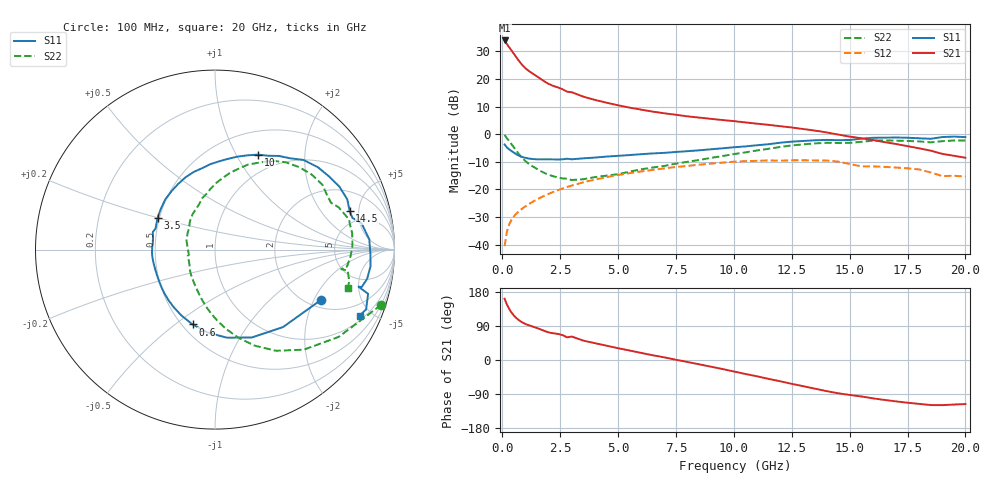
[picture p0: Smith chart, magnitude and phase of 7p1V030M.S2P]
! Infineon Technologies  Discrete & RF Semiconductors
! bfp620
! VCE =  1.0 V,  IC =  30 mA
! Common Emitter S-Parameters:  Sep 2002
# GHz  S  MA  R  50
!  f  S11  S21  S12  S22
! GHz  MAG  ANG  MAG  ANG  MAG  ANG  MAG  ANG
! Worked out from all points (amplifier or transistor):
!   59 points, 100 MHz to 20 GHz, reference 50 ohm
!   highest |S21| = 33.9 dB at 100 MHz (marker M1)
!   |S21| within 3 dB of that: start of sweep to 344.2 MHz
!   unconditionally stable (mu >= 1): 3.205 GHz to 9.953 GHz; 17.13 GHz to end of sweep
!   at 1 GHz: K = 0.78, MSG = 25.0 dB, |S12| = -26.1 dB
!   at 5.5 GHz: K = 1.04, MAG = 10.7 dB, |S12| = -14.1 dB
!   at 20 GHz: K = 1.39, MAG = -0.3 dB, |S12| = -15.3 dB
!   S11 on the Smith chart (normalised r, x): 100 MHz: 2.31, -2.26; 600 MHz: 0.56, -0.58; 3.5 GHz: 0.49, +0.20; 10 GHz: 0.77, +1.23; 14.5 GHz: 3.60, +3.96; 20 GHz: 1.25, -4.26
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0.1  0.6524 -25.6  49.83 161.6  0.0094 82.2  0.9759 -18.4
0.2  0.5745 -48.7  42.72 146.3  0.0173 70.1  0.8436 -35.2
0.3  0.531 -67.2  37.4 134.4  0.0234 65.0  0.7456 -48.4
0.4  0.4954 -82.3  32.77 125.0  0.0284 61.9  0.6584 -58.9
0.5  0.4631 -95.3  28.59 117.4  0.0325 59.7  0.578 -67.7
0.6  0.4351 -106.7  24.91 111.2  0.0362 58.2  0.5063 -75.3
0.7  0.4127 -116.7  21.79 105.9  0.0396 57.3  0.4453 -82.2
0.9  0.3828 -132.6  17.24 98.0  0.0462 56.3  0.3562 -93.6
1.1  0.3658 -143.9  14.45 92.6  0.0527 56.0  0.3009 -102.3
1.3  0.3559 -152.5  12.61 88.5  0.0594 55.6  0.2639 -109.5
2  0.3515 -177.3  8.154 72.9  0.0832 52.3  0.1846 -138.4
2.8  0.36 164.2  5.882 59.6  0.1109 46.6  0.1563 -166.7
3  0.3513 160.6  5.759 61.9  0.1177 44.9  0.1482 -168.6
3.5  0.3658 151.1  4.789 51.1  0.1347 40.4  0.153 176.1
5  0.4057 126.7  3.341 31.1  0.1826 26.1  0.1891 139.5
7  0.4598 98.7  2.391 6.9  0.2405 6.4  0.2664 109.6
10  0.5807 65.7  1.726 -30.3  0.3179 -26.8  0.4363 78.9
10.5  0.6014 60.4  1.636 -36.9  0.3254 -33.4  0.4689 73.8
13.5  0.7767 26.9  1.163 -75.6  0.3352 -69.2  0.6816 38.0
14.5  0.7803 16.0  0.986 -87.8  0.3195 -84.4  0.6941 25.6
17  0.8712 -6.2  0.665 -109.2  0.2492 -100.5  0.7656 1.4
20  0.886 -24.5  0.375 -116.2  0.1714 -111.0  0.7698 -16.1
